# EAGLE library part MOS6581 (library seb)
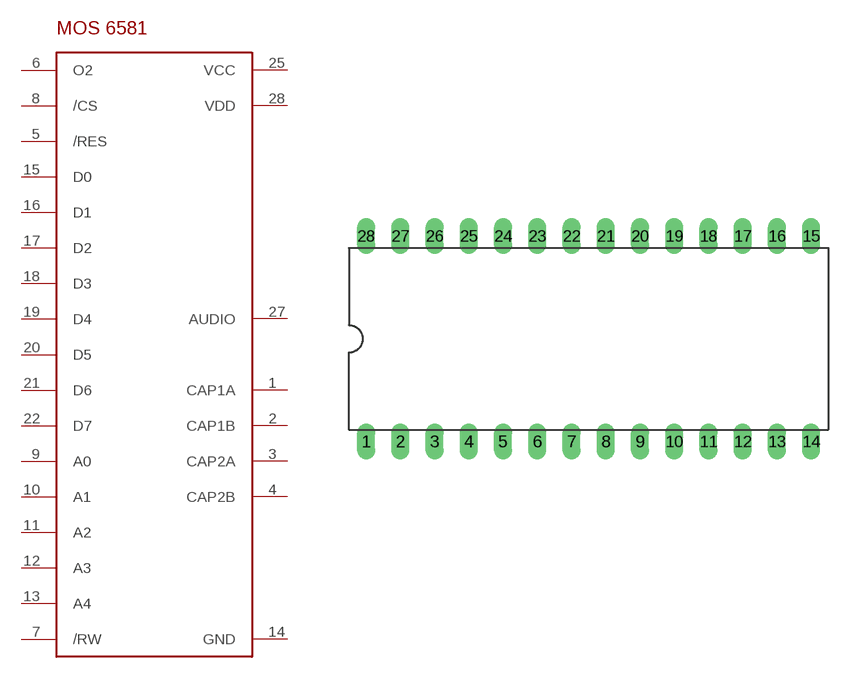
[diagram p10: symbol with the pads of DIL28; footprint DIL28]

Designator prefix IC

## MOS6581  [DIL28]
1  CAP1A
2  CAP1B
3  CAP2A
4  CAP2B
5  /RES
6  O2
7  /RW
8  /CS
9  A0
10  A1
11  A2
12  A3
13  A4
14  GND
15  D0
16  D1
17  D2
18  D3
19  D4
20  D5
21  D6
22  D7
25  VCC
27  AUDIO
28  VDD

## Footprint DIL28 (pad centres in mm)
Dual In Line Package
drill 0.813 long: 1 -16.51,-7.62; 2 -13.97,-7.62; 3 -11.43,-7.62; 4 -8.89,-7.62; 5 -6.35,-7.62; 6 -3.81,-7.62; 7 -1.27,-7.62; 8 1.27,-7.62; 9 3.81,-7.62; 10 6.35,-7.62; 11 8.89,-7.62; 12 11.43,-7.62; 13 13.97,-7.62; 14 16.51,-7.62; 15 16.51,7.62; 16 13.97,7.62; 17 11.43,7.62; 18 8.89,7.62; 19 6.35,7.62; 20 3.81,7.62; 21 1.27,7.62; 22 -1.27,7.62; 23 -3.81,7.62; 24 -6.35,7.62; 25 -8.89,7.62; 26 -11.43,7.62; 27 -13.97,7.62; 28 -16.51,7.62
